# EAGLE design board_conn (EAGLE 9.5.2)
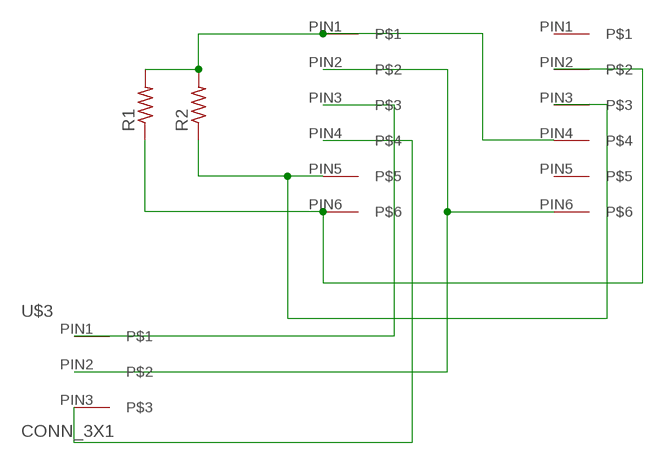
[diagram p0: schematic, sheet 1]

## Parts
R1  R1206FAB  [R1206FAB]
R2  R1206FAB  [R1206FAB]
U$1  CONN_6X1  [CONN_6X1]
U$2  CONN_6X1  [CONN_6X1]
U$3  CONN_3X1  [CONN_3X1]

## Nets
N$1: U$1.PIN2 U$2.PIN6 U$3.PIN2
N$3: R2.1 U$1.PIN5 U$2.PIN3
N$4: R1.1 U$1.PIN6 U$2.PIN2
N$5: R1.2 R2.2 U$1.PIN1 U$2.PIN4
N$7: U$1.PIN3 U$3.PIN1
N$8: U$1.PIN4 U$3.PIN3
Unconnected: U$2.PIN1 U$2.PIN5

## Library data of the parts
R1 R2 = fab:R: Resistor (US Symbol)
U$1 U$2 = ESP32-CAM:CONN_6X1
U$3 = ESP32-CAM:CONN_3X1

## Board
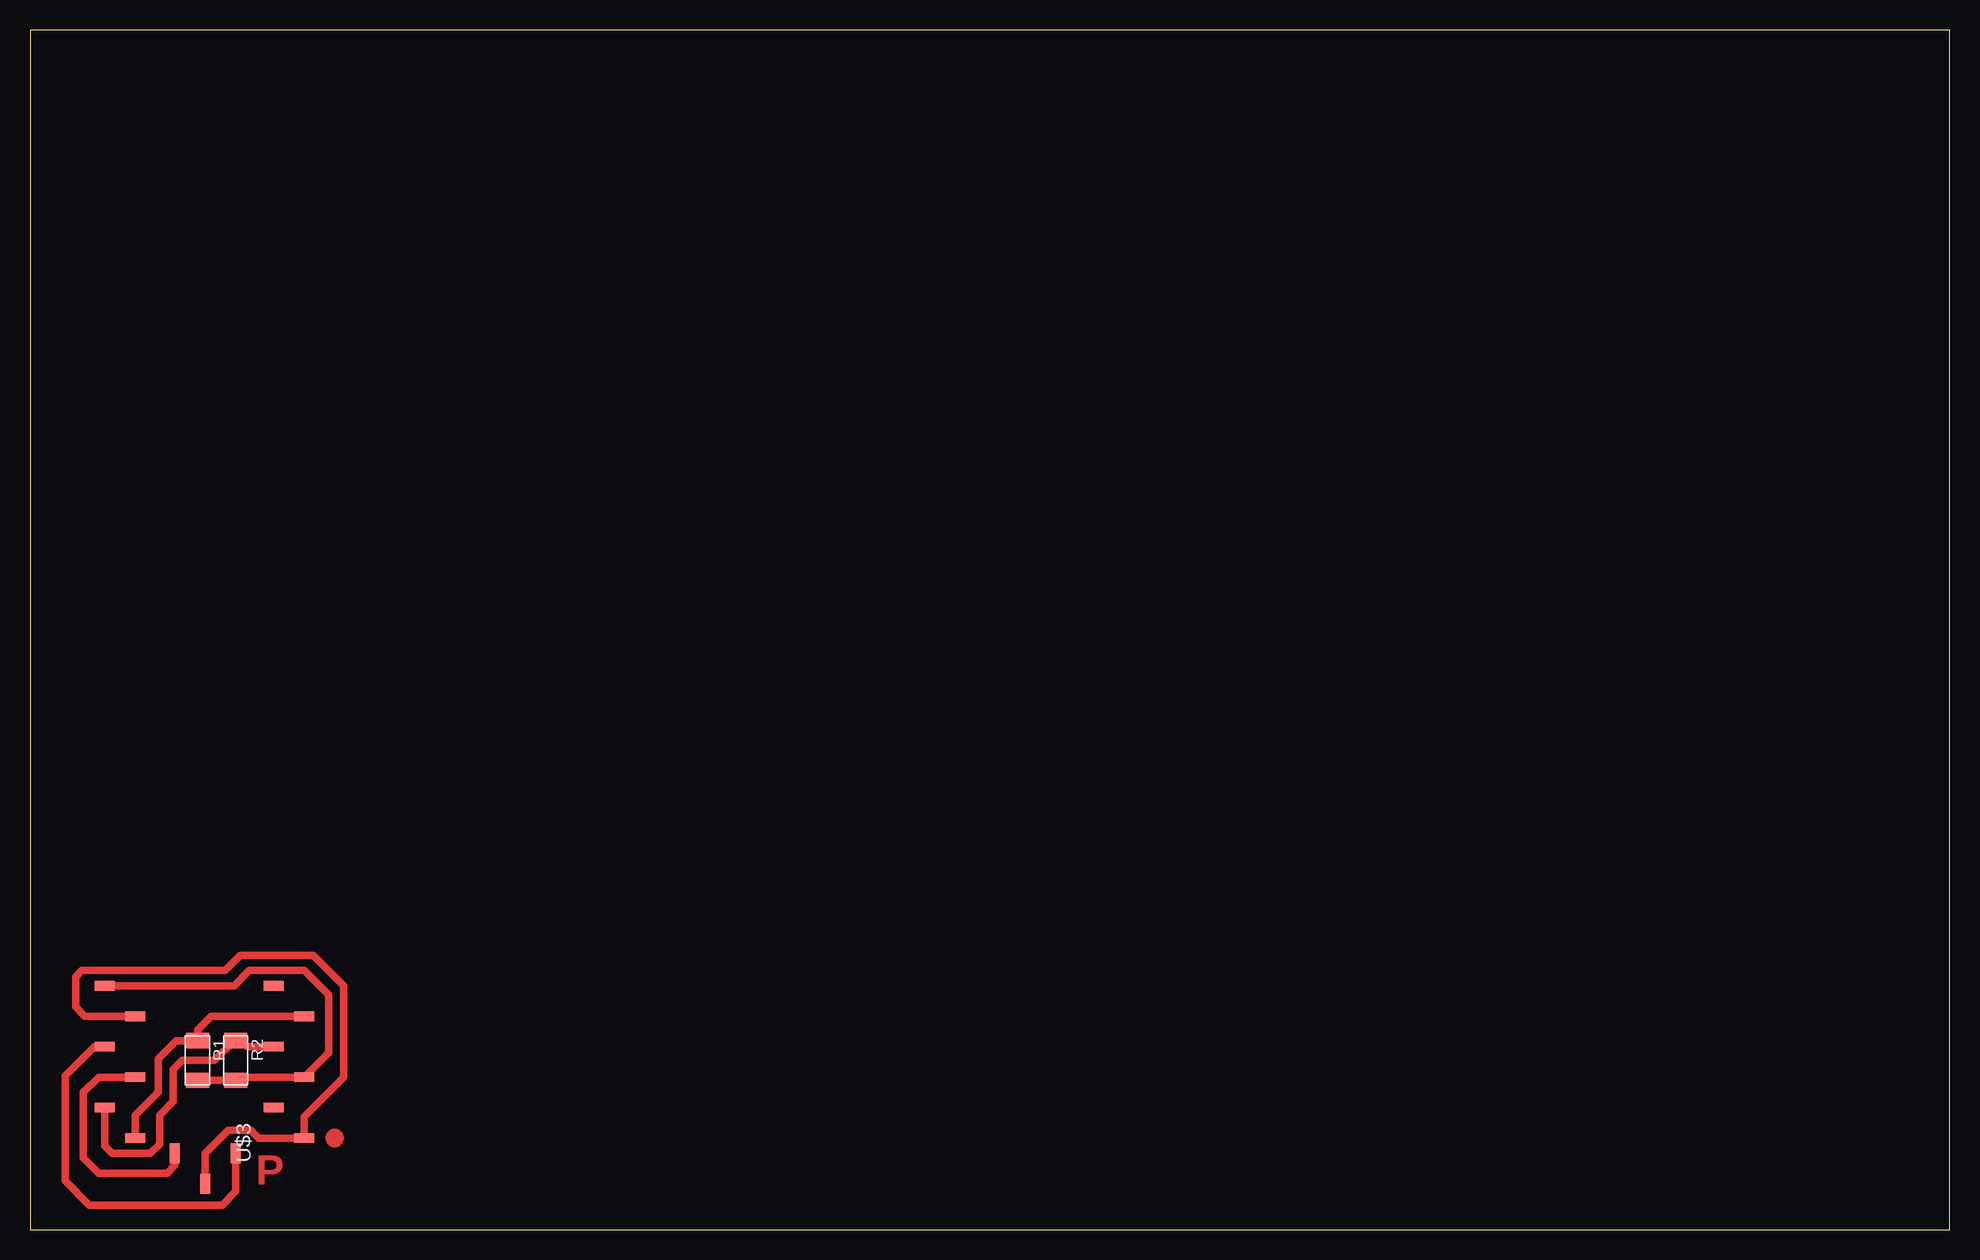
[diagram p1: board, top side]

Size 160 x 100 mm. Coordinates in mm from the lower left corner, seen from the top.
Outline: 0,0 160,0 160,100 0,100 0,0
Copper layers (1*16): Top 0.035mm / dielectric 1.5mm / Bottom 0.035mm
Design rules "default *": minimum track width 6mil, minimum drill 0.35mm, track to track 16mil, track to pad 16mil, pad to pad 16mil, via to via 16mil, smd to smd 16mil, copper to edge 40mil, drill to drill 6mil, minimum pad ring 10mil, minimum via ring 8mil, stop-mask expansion 4mil, vias tented up to drill 0mil, thermal gap 10mil

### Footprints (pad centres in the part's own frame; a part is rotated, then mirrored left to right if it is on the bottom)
R1206FAB = smd 1.27 x 1.905: 1 -1.651,0; 2 1.651,0
CONN_6X1 = smd 1.676 x 0.813: PIN1 -1.27,6.35; PIN2 1.27,3.81; PIN3 -1.27,1.27; PIN4 1.27,-1.27; PIN5 -1.27,-3.81; PIN6 1.27,-6.35
CONN_3X1 = smd 1.676 x 0.813: PIN1 -1.27,2.54; PIN2 1.27,0; PIN3 -1.27,-2.54

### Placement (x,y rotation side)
R1  13.97,14.1 270 top
R2  17.14,14.1 270 top
U$1  7.49,13.97 0 top
U$2  21.59,13.97 0 top
U$3  14.61,5.08 270 top

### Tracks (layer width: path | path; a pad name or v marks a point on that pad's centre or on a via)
N$1
  Top 0.61: U$3.PIN2 14.61,6.35 16.51,8.26 18.41,8.26 19.05,7.62 U$2.PIN6 22.86,9.4 26.16,12.7 26.16,20.32 23.62,22.86 17.53,22.86 16.26,21.59 4.32,21.59 3.81,21.08 3.81,18.54 4.57,17.78 U$1.PIN2
N$3
  Top 0.61: U$1.PIN5 6.22,6.99 6.86,6.35 10.03,6.35 10.79,7.11 10.79,9.53 11.94,10.67 11.94,13.34 12.7,14.1 15.37,14.1 17.02,15.75 R2.1 17.65,15.75 18.16,15.24 U$2.PIN3
N$4
  Top 0.61: U$1.PIN6 8.76,9.53 10.67,11.43 10.67,14.22 12.19,15.75 R1.1 13.97,16.64 15.11,17.78 U$2.PIN2
N$5
  Top 0.61: U$1.PIN1 17.02,20.32 18.29,21.59 22.86,21.59 24.89,19.56 24.89,14.73 U$2.PIN4 17.4,12.7 R2.2 R1.2
N$7
  Top 0.61: U$1.PIN3 5.33,15.24 2.92,12.83 2.92,4.06 4.95,2.03 16,2.03 17.14,3.17 U$3.PIN1
N$8
  Top 0.61: U$1.PIN4 5.71,12.7 4.45,11.43 4.45,5.97 5.71,4.7 11.43,4.7 12.06,5.33 U$3.PIN3
(copper drawn outside any net)
  shapes: Top circle x1

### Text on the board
Top: P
